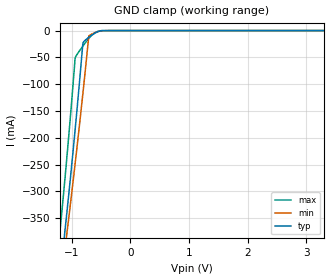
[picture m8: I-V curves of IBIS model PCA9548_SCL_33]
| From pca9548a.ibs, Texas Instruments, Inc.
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[Model]   PCA9548_SCL_33
Model_type  Terminator
| variable   typ   min   max
C_comp   7.25pF   5.60pF   9.50pF
| C_tri-state   7.25pF   5.60pF   9.50pF
[Temperature Range]   40   100   -40
| Ambient temperature   25   85   -40
[Voltage range]   3.3   3   3.6
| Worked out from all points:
|   GND clamp passes 1 mA (typ) near -0.52 V on its own axis
[GND Clamp]
| PCA9548_SCL_33
|   Voltage   I(typ)   I(min)   I(max)
-5.5V     -3.656A    -3.511A    -3.814A
-1.215V   -469.9mA   -491.5mA   -387.7mA
-1.17V    -425.8mA   -453mA     -337mA
-1.125V   -380.5mA   -413.8mA   -284.5mA
-1.1V     -354.8mA   -391.7mA   -254.5mA
-1.075V   -328.7mA   -369.3mA   -223.8mA
-945mV    -185.6mA   -249mA     -52.16mA
-810mV    -22.62mA   -115.3mA   -28.77mA
-715mV    -12.8mA    -14.19mA   -15.21mA
-695mV    -11.15mA   -8.703mA   -12.71mA
-490mV    -200.7uA   -350.6uA   -29.52uA
3.3V      308.2pA    829.7pA    194pA
